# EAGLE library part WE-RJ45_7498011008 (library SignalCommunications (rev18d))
Order Code 7498011008 Design SMD xBase-T 10/100 Base-T Ports 1x1 Application Standard Tab Position Down LED (Left-Right) None EMI Fingers Yes Details see: http://katalog.we-online.de/en/pbs/WE-LAN_RJ45/7498011008? Updated by Yingchun Shan 2016-08-23 2014 (C) Würth Elektronik
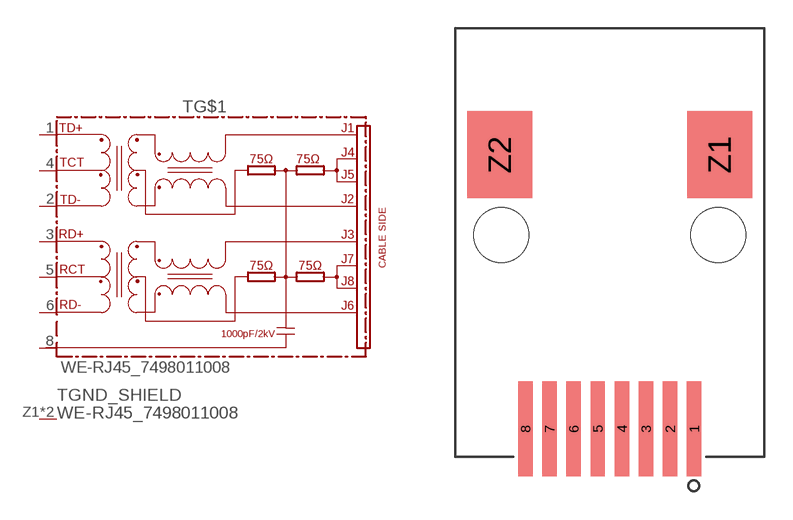
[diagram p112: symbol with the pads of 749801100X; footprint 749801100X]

Designator prefix T; gates GND_SHIELD=GND_PIN G$1=74990X-THT-10/100-T

## WE-RJ45_7498011008 (COMPANY-URL: http://www.we-online.de; CREATED-BY: Christin Zierenner; CREATED-DATE: AUG 2012; DATASHEET-URL: http://katalog.we-online.de/kataloge/eisos/media/pdf/7498011008.pdf; MANUFACTURER: Würth Elektronik eiSos GmbH)  [749801100X]
1  G$1:TD+
2  G$1:TD-
3  G$1:RD+
4  G$1:TCT
5  G$1:RCT
6  G$1:RD-
8  G$1:8
Z1  GND_SHIELD:1  pwr
Z2  GND_SHIELD:1  pwr

## Footprint 749801100X (pad centres in mm)
MAX HEIGHT=13.60mm PORTS----1X1 LED --No
smd 0.76 x 5: 1 4.445,-10.2; 2 3.175,-10.2; 3 1.905,-10.2; 4 0.635,-10.2; 5 -0.635,-10.2; 6 -1.905,-10.2; 7 -3.175,-10.2; 8 -4.445,-10.2
smd 3.42 x 4.58: Z1 5.79,4.24; Z2 -5.79,4.24
hole 2.9 at -5.715,0
hole 2.9 at 5.715,0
